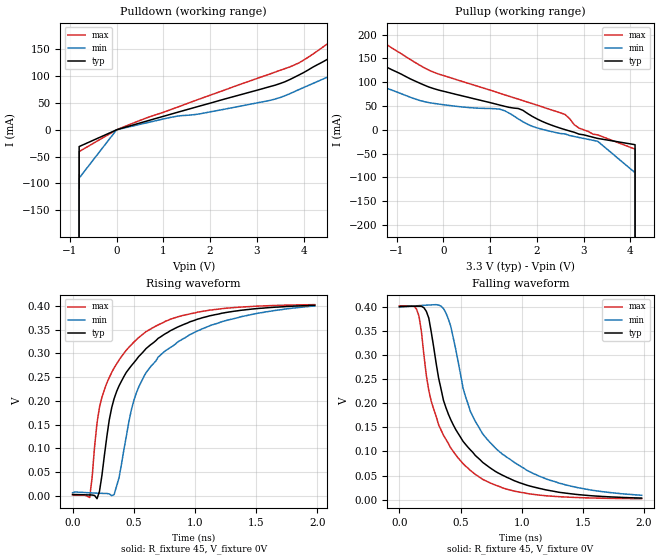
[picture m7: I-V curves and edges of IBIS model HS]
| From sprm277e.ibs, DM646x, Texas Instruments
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|   0.00000035   8.46100mV   16.75000mV   6.76600mV
[Model] HS
Model_type Output
Polarity Non-Inverting
Cref = 0.001pF
Rref = 45
Vref = 0V
Vmeas =0.2V
| typ min max
C_comp 2.0pF NA NA
|Voh = 0.3V
|Vol = 0.075V
|[Model Spec]
| typ min max
| typ min max
|Voh 0.7V 0.3V 1.15V
|Vol 0.01V -0.3V 0.075V
[Temperature Range] 25 125 -40
[Voltage Range] 3.30V 3.0V 3.6V
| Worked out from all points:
|   slope of the pulldown table from 0 to 0.495 V, typ, clamps not added: 39.2 ohm
|   slope of the pullup table from 0 to 0.495 V, typ, clamps not added: 41.5 ohm
|   rising waveform, R_fixture 45, V_fixture 0V: 20-80 % time 397ps typ, 435ps min, 323ps max; typ from 0.003 V to 0.401 V
|   falling waveform, R_fixture 45, V_fixture 0V: 20-80 % time 382ps typ, 430ps min, 305ps max; typ from 0.401 V to 0.003 V
| (Vdd votage range) 1.50V 1.35V 1.65V
| (Process strength) nominal weak strong
[Pulldown]
-3.3V     -393A      -305A      -455A
-800mV    -31.2mA    -90mA      -40.5mA
0V        0A         0A         0A
1.2V      30.14mA    23.98mA    39.06mA
1.8V      44.87mA    30.07mA    58.28mA
3.3V      81.08mA    55.27mA    104.8mA
3.8V      97.81mA    71mA       120.8mA
4.1V      111.7mA    82.64mA    135.3mA
5V        155.1mA    117.6mA    190.8mA
5.7V      189.5mA    144.6mA    235.4mA
6.3V      219.5mA    169mA      272.3mA
6.6V      234mA      169mA      291.5mA
[Pullup]
-3.3V     234mA      169mA      310mA
-2.9V     215mA      153mA      285mA
-1.8V     160.2mA    110mA      216mA
-300mV    89.56mA    56.97mA    124.8mA
1.2V      52.16mA    43.47mA    77.03mA
1.6V      44.85mA    23.03mA    64.55mA
1.9V      28.35mA    7.49mA     55.13mA
2.6V      461.5uA    -8.541mA   32.44mA
2.9V      -9mA       -16.05mA   3.697mA
3.3V      -18mA      -24mA      -10.59mA
4.1V      -31.2mA    -90mA      -40.5mA
6.6V      -393A      -305A      -455A
[Ramp]
| variable typ min max
dV/dt_r 0.228837V/0.397254ns 0.245233V/0.437455ns 0.240251V/0.323073ns
dV/dt_f 0.228856V/0.382777ns 0.245259V/0.43228ns 0.240342V/0.304743ns
R_load = 45
[Rising Waveform]
R_fixture = 45
V_fixture = 0V
V_fixture_min = 0V
V_fixture_max = 0V
0s        3.03mV     6.68mV     1.982mV
140ps     2.05mV     6.57mV     -3.239mV
200ps     -5.8mV     5.81mV     153.4mV
240ps     42.97mV    5.39mV     207.1mV
300ps     159.9mV    4.36mV     248.8mV
340ps     204.9mV    2.92mV     269.5mV
480ps     273.7mV    180.3mV    317.8mV
600ps     309.7mV    259mV      345.4mV
1.12ns    378.8mV    357.9mV    390.7mV
1.98ns    400.9mV    399.5mV    402.3mV
|   0.000000002   0.40100   0.40000   0.40240V
[Falling Waveform]
R_fixture = 45
V_fixture = 0V
V_fixture_min = 0V
V_fixture_max = 0V
0s        401mV      400mV      402.4mV
140ps     401.8mV    402.6mV    395.6mV
180ps     401.7mV    403.3mV    348.3mV
220ps     391.1mV    403.9mV    257.7mV
360ps     206.2mV    396.9mV    133.7mV
420ps     165.7mV    359.5mV    107mV
580ps     103.2mV    183.3mV    60.42mV
780ps     59.3mV     108.3mV    30.53mV
1.1ns     25.92mV    53.34mV    10.66mV
1.98ns    3.138mV    8.921mV    1.857mV
